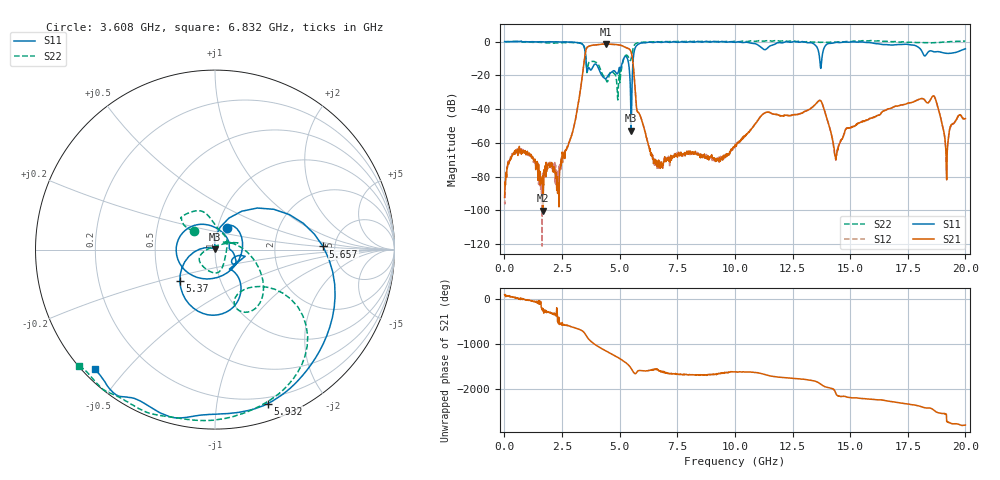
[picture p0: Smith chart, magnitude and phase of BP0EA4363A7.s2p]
! 9/17/2020 12:55:40 PM
! C:\ANRITSUVNA\DATA\MLO\SAMPLES\RAYTHEOM BP\17375_20GH_91720 .S2P
! CHANNEL.1
! TR.MEASUREMENT
! CORRECTED.DATA
# GHZ S RI R 50.0
! FREQ.GHZ  S11RE  S11IM  S31RE  S31IM  S13RE  S13IM  S33RE  S33IM
!; PortSelection: Port_13
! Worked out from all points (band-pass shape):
!   1601 points, 10 MHz to 20 GHz, reference 50 ohm
!   highest |S21| = -1.49 dB at 4.42 GHz (marker M1); lowest = -100.3 dB at 1.684 GHz (marker M2)
!   |S21| within 3 dB of the highest: 3.551 GHz to 5.424 GHz (1.873 GHz wide, 41.7 % of centre)
!   lowest |S11| = -52.8 dB at 5.495 GHz (marker M3), VSWR 1.00, Z = 50.2 + j0.111 ohm
!   |S11| at or under -10 dB: 3.536 GHz to 5.176 GHz (1.64 GHz wide, 37.7 % of centre); 5.337 GHz to 5.592 GHz (255.8 MHz wide, 4.68 % of centre); 13.68 GHz to 13.77 GHz (98.19 MHz wide, 0.715 % of centre)
!   |S22| runs from -34.6 to 0.7 dB; largest |S21 - S12| = 0.0021
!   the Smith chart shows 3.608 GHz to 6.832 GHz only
!   S11 on the Smith chart (normalised r, x): 3.608 GHz: 1.11, +0.28; 5.37 GHz: 0.64, -0.24; 5.657 GHz: 4.01, +0.22; 5.932 GHz: 0.14, -1.39; 6.832 GHz: 0.03, -0.41
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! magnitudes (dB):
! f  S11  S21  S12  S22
! 10 MHz  0.0  -92.5  -95.3  0.0
! 697.2 MHz  0.1  -65.3  -64.6  0.2
! 1.684 GHz  -0.2  -100.3  -87.8  -0.5
! 2.359 GHz  -0.2  -91.2  -76.9  -0.8
! 3.346 GHz  -1.2  -24.1  -24.0  -1.1
! 3.608 GHz  -17.1  -3.2  -3.2  -16.0
! 4.42 GHz  -21.8  -1.5  -1.5  -23.0
! 5.37 GHz  -11.6  -4.0  -4.0  -8.9
! 5.495 GHz  -52.8  -6.1  -6.1  -10.5
! 5.657 GHz  -4.4  -25.2  -25.2  -1.7
! 5.932 GHz  -0.8  -45.4  -45.3  -0.4
! 6.682 GHz  -0.2  -74.2  -75.1  -0.1
! 6.832 GHz  -0.5  -72.7  -73.5  0.0
! 10.01 GHz  -0.4  -61.8  -61.8  0.2
! 11.32 GHz  -4.8  -42.2  -42.2  0.4
! 13.34 GHz  -0.8  -39.1  -39.1  -0.3
! 13.77 GHz  -11.1  -36.0  -36.0  -0.4
! 14.39 GHz  -0.4  -68.8  -68.8  -0.4
! 16.68 GHz  -1.9  -39.9  -39.7  0.1
! 18.63 GHz  -6.0  -32.2  -32.2  -0.6
! 19.19 GHz  -7.0  -82.0  -77.3  -0.2
! 20 GHz  -4.3  -45.6  -45.7  0.4
